| IBIS file stm32f7x2_lqfp100.ibs
[IBIS ver] 4.2
[File name] stm32f7x2_lqfp100.ibs
[File Rev] 1.1
[Date]  21-12-2016
[Source] Data Created at STMicroelectronics
[Notes]  File originated from ELDO simulations.
[Disclaimer]  This information is for modeling purpose only and is
   not guaranted.
   The information is subject to change without notice.
[Copyright] Copyright 2017 STMicroelectronics Inc.
|   Component stm32f7x2_lqfp100
[Component] stm32f7x2_lqfp100
[Manufacturer] STMicroelectronics
[Package]
| variable   typ   min   max
R_pkg   0.0   0.0   0.0
L_pkg   0.0H   0.0H   0.0H
C_pkg   0.0F   0.0F   0.0F
[Pin]  signal_name   model_name   R_pin   L_pin   C_pin
1 PE2 io8p_arsudq_ft 132.430E-3 7.034E-9 135.000E-15
2 PE3 io8p_arsudq_ft 133.348E-3 6.765E-9 19.500E-15
3 PE4 io8p_arsudq_ft 128.973E-3 6.495E-9 10.400E-15
4 PE5 io8p_arsudq_ft 125.345E-3 6.206E-9 5.240E-15
5 PE6 io8p_arsudq_ft 120.515E-3 5.991E-9 7.820E-15
6 VBAT power 120.471E-3 5.950E-9 6.530E-15
7 PC13 io8p_arwsudq_ft_v33 117.881E-3 5.783E-9 6.230E-15
8 PC14-OSC32_IN io8p_arwsudq_ft_v33 117.279E-3 5.654E-9 3.110E-15
9 PC15-OSC32_OUT io8p_arwsudq_ft 115.548E-3 5.548E-9 1.390E-15
10 VSS gnd 114.996E-3 5.434E-9 2.920E-15
11 VDD power 112.976E-3 5.296E-9 3.560E-15
12 PH0-OSC_IN io8p_arsudq_ft 111.323E-3 5.231E-9 4.780E-15
13 PH1-OSC_OUT io8p_arsudq_ft 109.217E-3 5.142E-9 8.660E-15
14 NRST ioreset_ft_v33 110.664E-3 5.180E-9 9.030E-15
15 PC0 io8p_ar3wsudq_ft 110.608E-3 5.192E-9 7.980E-15
16 PC1 io8p_ar3wsudq_ft_v33 111.326E-3 5.252E-9 10.300E-15
17 PC2 io8p_ar3wsudq_ft 114.420E-3 5.345E-9 7.000E-15
18 PC3 io8p_ar3wsudq_ft 114.363E-3 5.454E-9 8.650E-15
19 VSSA gnd 117.564E-3 5.621E-9 7.825E-15
20 VREF+ power 119.905E-3 5.800E-9 229.000E-18
21 VDDA power 122.312E-3 5.963E-9 1.050E-15
22 PA0-WKUP io8p_ar3wsudq_ft_v33 125.384E-3 6.187E-9 812.000E-18
23 PA1 io8p_ar3wsudq_ft 129.702E-3 6.485E-9 3.820E-15
24 PA2 io8p_ar3wsudq_ft_v33 132.290E-3 6.715E-9 6.800E-15
25 PA3 io8p_ar3wsudq_ft 132.955E-3 7.014E-9 16.700E-15
26 VSS gnd 133.943E-3 7.050E-9 17.500E-15
27 VDD power 134.958E-3 6.804E-9 12.700E-15
28 PA4 io8p_ar3wsudq_ft 130.511E-3 6.528E-9 9.830E-15
29 PA5 io8p_ar3wsudq_ft 125.387E-3 6.245E-9 6.070E-15
30 PA6 io8p_ar3wsudq_ft 124.989E-3 6.108E-9 577.000E-18
31 PA7 io8p_ar3wsudq_ft 121.784E-3 5.890E-9 1.520E-15
32 PC4 io8p_ar3wsudq_ft 119.149E-3 5.716E-9 5.440E-15
33 PC5 io8p_ar3wsudq_ft 116.375E-3 5.556E-9 4.100E-15
34 PB0 io8p_ar3wsudq_ft 113.279E-3 5.415E-9 3.690E-15
35 PB1 io8p_ar3wsudq_ft 112.727E-3 5.358E-9 3.895E-15
36 PB2 io8p_ar3wsudq_ft 112.271E-3 5.272E-9 1.660E-15
37 PE7 io8p_arsudq_ft 111.816E-3 5.238E-9 7.920E-15
38 PE8 io8p_arsudq_ft 110.999E-3 5.184E-9 9.900E-15
39 PE9 io8p_arsudq_ft 114.589E-3 5.299E-9 7.910E-15
40 PE10 io8p_arsudq_ft 114.461E-3 5.333E-9 7.940E-15
41 PE11 io8p_arsudq_ft 115.350E-3 5.424E-9 4.180E-15
42 PE12 io8p_arsudq_ft 116.979E-3 5.533E-9 6.060E-15
43 PE13 io8p_arsudq_ft 120.185E-3 5.698E-9 5.120E-15
44 PE14 io8p_arsudq_ft 122.587E-3 5.871E-9 4.740E-15
45 PE15 io8p_ar3wsudq_ft 126.303E-3 6.069E-9 11.600E-15
46 PB10 io8p_arsudq_i2c_ft 129.715E-3 6.277E-9 9.910E-15
47 PB11 io8p_arsudq_i2c_ft 133.373E-3 6.508E-9 5.080E-15
48 VCAP_1 power 137.888E-3 6.857E-9 5.470E-15
49 VSS gnd 131.554E-3 6.802E-9 4.180E-15
50 VDD power 132.348E-3 7.042E-9 11.900E-15
51 PB12 io8usb_id_otg_ft 131.768E-3 7.008E-9 16.200E-15
52 PB13 io8usb_vbus_otg_ft 131.784E-3 6.751E-9 2.150E-15
53 PB14 io8usb_lsfs_otg_ft 129.151E-3 6.483E-9 9.175E-15
54 PB15 io8usb_lsfs_otg_ft 125.191E-3 6.202E-9 5.663E-15
55 PD8 io8p_arsudq_ft 121.530E-3 5.986E-9 3.690E-15
56 PD9 io8p_arsudq_ft 118.874E-3 5.807E-9 7.430E-15
57 PD10 io8p_arsudq_ft 115.870E-3 5.635E-9 10.600E-15
58 PD11 io8p_arsudq_ft 113.226E-3 5.471E-9 5.760E-15
59 PD12 io8p_arsudq_ft 111.782E-3 5.354E-9 6.530E-15
60 PD13 io8p_arsudq_ft 110.713E-3 5.276E-9 11.400E-15
61 PD14 io8p_arsudq_ft 110.052E-3 5.204E-9 13.200E-15
62 PD15 io8p_arsudq_ft 109.954E-3 5.180E-9 14.600E-15
63 PC6 io8p_arsudq_ft 109.780E-3 5.154E-9 7.250E-15
64 PC7 io8p_arsudq_ft 112.446E-3 5.258E-9 359.000E-18
65 PC8 io8p_arsudq_ft 113.596E-3 5.332E-9 658.000E-18
66 PC9 io8p_arsudq_i2c_ft 115.707E-3 5.466E-9 508.500E-18
67 PA8 io8p_arsudq_i2c_ft 116.952E-3 5.598E-9 583.250E-18
68 PA9 io8usb_vbus_otg_ft 119.043E-3 5.762E-9 545.875E-18
69 PA10 io8usb_id_otg_ft 120.674E-3 5.880E-9 13.900E-15
70 PA11 io8usb_lsfs_otg_ft 124.659E-3 6.108E-9 25.000E-15
71 PA12 io8usb_lsfs_otg_ft 124.407E-3 6.161E-9 39.900E-15
72 PA13 io8p_arsudq_ft 130.156E-3 6.404E-9 302.000E-15
73 VCAP_2 power 135.110E-3 6.824E-9 155.000E-15
74 VSS gnd 139.402E-3 7.077E-9 155.000E-15
75 VDD power 133.554E-3 7.056E-9 39.000E-15
76 PA14 io8p_arsudq_ft 135.295E-3 7.104E-9 16.300E-15
77 PA15 io8p_arsudq_ft 132.514E-3 6.836E-9 9.760E-15
78 PC10 io8p_arsudq_ft 133.482E-3 6.641E-9 9.300E-15
79 PC11 io8p_arsudq_ft 128.366E-3 6.341E-9 5.420E-15
80 PC12 io8p_arsudq_ft 124.282E-3 6.092E-9 1.180E-15
81 PD0 io8p_arsudq_ft 121.841E-3 5.917E-9 5.460E-15
82 PD1 io8p_arsudq_ft 118.487E-3 5.728E-9 7.000E-15
83 PD2 io8p_arsudq_ft 117.180E-3 5.573E-9 6.060E-15
84 PD3 io8p_arsudq_ft 113.501E-3 5.422E-9 5.450E-15
85 PD4 io8p_arsudq_ft 113.789E-3 5.344E-9 529.000E-18
86 PD5 io8p_arsudq_ft 110.806E-3 5.256E-9 2.990E-15
87 PD6 io8p_arsudq_ft 110.442E-3 5.246E-9 2.060E-15
88 PD7 io8p_arsudq_ft 111.525E-3 5.178E-9 5.680E-15
89 PB3 io8p_arsudq_ft 111.144E-3 5.223E-9 9.910E-15
90 PB4 io8p_arsudq_ft 113.222E-3 5.310E-9 9.050E-15
91 PB5 io8p_ar3wsudq_ft 113.323E-3 5.401E-9 12.900E-15
92 PB6 io8p_arsudq_i2c_ft 115.849E-3 5.519E-9 12.600E-15
93 PB7 io8p_arsudq_i2c_ft 117.578E-3 5.673E-9 6.140E-15
94 BOOT0 vpp_test_hv 118.982E-3 5.802E-9 9.370E-15
95 PB8 io8p_arsudq_i2c_ft 121.886E-3 5.962E-9 7.755E-15
96 PB9 io8p_arsudq_i2c_ft 126.276E-3 6.158E-9 8.563E-15
97 PE0 io8p_arsudq_ft 128.749E-3 6.367E-9 8.159E-15
98 PE1 io8p_arsudq_ft 133.288E-3 6.700E-9 1.030E-15
99 VSS gnd 132.230E-3 6.844E-9 4.410E-15
100 VDD power 132.277E-3 7.052E-9 17.100E-15
[Diff Pin]   inv_pin   vdiff   tdelay_typ  tdelay_min  tdelay_max
53   54   NA   NA   NA   NA
70   71   NA   NA   NA   NA
[Model Selector] io8p_ar3wsudq_ft
io8p00_ar3wsudq_ft_pd_lv  "SPEED00 1P8V, PD=40kOhm"
io8p00_ar3wsudq_ft_pu_lv  "SPEED00 1P8V, PU=40kOhm"
io8p00_ar3wsudq_ft_lv  "SPEED00 1P8V"
io8p01_ar3wsudq_ft_pd_lv  "SPEED01 1P8V, PD=40kOhm"
io8p01_ar3wsudq_ft_pu_lv  "SPEED01 1P8V, PU=40kOhm"
io8p01_ar3wsudq_ft_lv  "SPEED01 1P8V"
io8p10_ar3wsudq_ft_pd_lv  "SPEED10 1P8V, PD=40kOhm"
io8p10_ar3wsudq_ft_pu_lv  "SPEED10 1P8V, PU=40kOhm"
io8p10_ar3wsudq_ft_lv  "SPEED10 1P8V"
io8p11_ar3wsudq_ft_pd_lv  "SPEED11 1P8V, PD=40kOhm"
io8p11_ar3wsudq_ft_pu_lv  "SPEED11 1P8V, PU=40kOhm"
io8p11_ar3wsudq_ft_lv  "SPEED11 1P8V"
io8p00_ar3wsudq_ft_pd  "SPEED00, PD=40kOhm"
io8p00_ar3wsudq_ft_pu  "SPEED00, PU=40kOhm"
io8p00_ar3wsudq_ft  "SPEED00"
io8p01_ar3wsudq_ft_pd  "SPEED01, PD=40kOhm"
io8p01_ar3wsudq_ft_pu  "SPEED01, PU=40kOhm"
io8p01_ar3wsudq_ft  "SPEED01"
io8p10_ar3wsudq_ft_pd  "SPEED10, PD=40kOhm"
io8p10_ar3wsudq_ft_pu  "SPEED10, PU=40kOhm"
io8p10_ar3wsudq_ft  "SPEED10"
io8p11_ar3wsudq_ft_pd  "SPEED11, PD=40kOhm"
io8p11_ar3wsudq_ft_pu  "SPEED11, PU=40kOhm"
io8p11_ar3wsudq_ft  "SPEED11"
[Model Selector] io8p_ar3wsudq_ft_v33
io8p00_ar3wsudq_ft_v33_pd_lv  "SPEED00 1P8V, PD=40kOhm"
io8p00_ar3wsudq_ft_v33_pu_lv  "SPEED00 1P8V, PU=40kOhm"
io8p00_ar3wsudq_ft_v33_lv  "SPEED00 1P8V"
io8p01_ar3wsudq_ft_v33_pd_lv  "SPEED01 1P8V, PD=40kOhm"
io8p01_ar3wsudq_ft_v33_pu_lv  "SPEED01 1P8V, PU=40kOhm"
io8p01_ar3wsudq_ft_v33_lv  "SPEED01 1P8V"
io8p10_ar3wsudq_ft_v33_pd_lv  "SPEED10 1P8V, PD=40kOhm"
io8p10_ar3wsudq_ft_v33_pu_lv  "SPEED10 1P8V, PU=40kOhm"
io8p10_ar3wsudq_ft_v33_lv  "SPEED10 1P8V"
io8p11_ar3wsudq_ft_v33_pd_lv  "SPEED11 1P8V, PD=40kOhm"
io8p11_ar3wsudq_ft_v33_pu_lv  "SPEED11 1P8V, PU=40kOhm"
io8p11_ar3wsudq_ft_v33_lv  "SPEED11 1P8V"
io8p00_ar3wsudq_ft_v33_pd  "SPEED00, PD=40kOhm"
io8p00_ar3wsudq_ft_v33_pu  "SPEED00, PU=40kOhm"
io8p00_ar3wsudq_ft_v33  "SPEED00"
io8p01_ar3wsudq_ft_v33_pd  "SPEED01, PD=40kOhm"
io8p01_ar3wsudq_ft_v33_pu  "SPEED01, PU=40kOhm"
io8p01_ar3wsudq_ft_v33  "SPEED01"
io8p10_ar3wsudq_ft_v33_pd  "SPEED10, PD=40kOhm"
io8p10_ar3wsudq_ft_v33_pu  "SPEED10, PU=40kOhm"
io8p10_ar3wsudq_ft_v33  "SPEED10"
io8p11_ar3wsudq_ft_v33_pd  "SPEED11, PD=40kOhm"
io8p11_ar3wsudq_ft_v33_pu  "SPEED11, PU=40kOhm"
io8p11_ar3wsudq_ft_v33  "SPEED11"
[Model Selector] io8p_arsudq_ft
io8p00_arsudq_ft_pd_lv  "SPEED00 1P8V, PD=40kOhm"
io8p00_arsudq_ft_pu_lv  "SPEED00 1P8V, PU=40kOhm"
io8p00_arsudq_ft_lv  "SPEED00 1P8V"
io8p01_arsudq_ft_pd_lv  "SPEED01 1P8V, PD=40kOhm"
io8p01_arsudq_ft_pu_lv  "SPEED01 1P8V, PU=40kOhm"
io8p01_arsudq_ft_lv  "SPEED01 1P8V"
io8p10_arsudq_ft_pd_lv  "SPEED10 1P8V, PD=40kOhm"
io8p10_arsudq_ft_pu_lv  "SPEED10 1P8V, PU=40kOhm"
io8p10_arsudq_ft_lv  "SPEED10 1P8V"
io8p11_arsudq_ft_pd_lv  "SPEED11 1P8V, PD=40kOhm"
io8p11_arsudq_ft_pu_lv  "SPEED11 1P8V, PU=40kOhm"
io8p11_arsudq_ft_lv  "SPEED11 1P8V"
io8p00_arsudq_ft_pd  "SPEED00, PD=40kOhm"
io8p00_arsudq_ft_pu  "SPEED00, PU=40kOhm"
io8p00_arsudq_ft  "SPEED00"
io8p01_arsudq_ft_pd  "SPEED01, PD=40kOhm"
io8p01_arsudq_ft_pu  "SPEED01, PU=40kOhm"
io8p01_arsudq_ft  "SPEED01"
io8p10_arsudq_ft_pd  "SPEED10, PD=40kOhm"
io8p10_arsudq_ft_pu  "SPEED10, PU=40kOhm"
io8p10_arsudq_ft  "SPEED10"
io8p11_arsudq_ft_pd  "SPEED11, PD=40kOhm"
io8p11_arsudq_ft_pu  "SPEED11, PU=40kOhm"
io8p11_arsudq_ft  "SPEED11"
[Model Selector] io8p_arsudq_i2c_ft
io8prog_1v8_i2c_pd  "5V Tol GPIO 1.8V range i2c functionality with pull down"
io8prog_1v8_i2c_pu  "5V Tol GPIO 1.8V range i2c functionality with pull up"
io8prog_1v8_i2c  "5V Tol GPIO 1.8V range i2c functionality"
io8prog_3v3_i2c_pd  "5V Tol GPIO 3.3V range i2c functionality with pull down"
io8prog_3v3_i2c_pu  "5V Tol GPIO 3.3V range i2c functionality with pull up"
io8prog_3v3_i2c  "5V Tol GPIO 3.3V range i2c functionality"
io8prog_1v8_pd_00  "5V Tol GPIO 1.8V range with pd speed 00"
io8prog_1v8_pu_00  "5V Tol GPIO 1.8V range with pu speed 00"
io8prog_1v8_00  "5V Tol GPIO 1.8V range speed 00"
io8prog_3v3_pd_00  "5V Tol GPIO 3.3V range with pd speed 00"
io8prog_3v3_pu_00  "5V Tol GPIO 3.3V range with pu speed 00"
io8prog_3v3_00  "5V Tol GPIO 3.3V range speed 00"
io8prog_1v8_pd_01  "5V Tol GPIO 1.8V range with pd speed 01"
io8prog_1v8_pu_01  "5V Tol GPIO 1.8V range with pu speed 01"
io8prog_1v8_01  "5V Tol GPIO 1.8V range speed 01"
io8prog_3v3_pd_01  "5V Tol GPIO 3.3V range with pd speed 01"
io8prog_3v3_pu_01  "5V Tol GPIO 3.3V range with pu speed 01"
io8prog_3v3_01  "5V Tol GPIO 3.3V range speed 01"
io8prog_1v8_pd_10  "5V Tol GPIO 1.8V range with pd speed 10"
io8prog_1v8_pu_10  "5V Tol GPIO 1.8V range with pu speed 10"
io8prog_1v8_10  "5V Tol GPIO 1.8V range speed 10"
io8prog_3v3_pd_10  "5V Tol GPIO 3.3V range with pd speed 10"
io8prog_3v3_pu_10  "5V Tol GPIO 3.3V range with pu speed 10"
io8prog_3v3_10  "5V Tol GPIO 3.3V range speed 10"
io8prog_1v8_pd_11  "5V Tol GPIO 1.8V range with pd speed 11"
io8prog_1v8_pu_11  "5V Tol GPIO 1.8V range with pu speed 11"
io8prog_1v8_11  "5V Tol GPIO 1.8V range speed 11"
io8prog_3v3_pd_11  "5V Tol GPIO 3.3V range with pd speed 11"
io8prog_3v3_pu_11  "5V Tol GPIO 3.3V range with pu speed 11"
io8prog_3v3_11  "5V Tol GPIO 3.3V range speed 11"
[Model Selector] io8p_arwsudq_ft
io8p00_arwsudq_ft_pd_lv  "SPEED00 1P8V, PD=40kOhm"
io8p00_arwsudq_ft_pu_lv  "SPEED00 1P8V, PU=40kOhm"
io8p00_arwsudq_ft_lv  "SPEED00 1P8V"
io8p01_arwsudq_ft_pd_lv  "SPEED01 1P8V, PD=40kOhm"
io8p01_arwsudq_ft_pu_lv  "SPEED01 1P8V, PU=40kOhm"
io8p01_arwsudq_ft_lv  "SPEED01 1P8V"
io8p10_arwsudq_ft_pd_lv  "SPEED10 1P8V, PD=40kOhm"
io8p10_arwsudq_ft_pu_lv  "SPEED10 1P8V, PU=40kOhm"
io8p10_arwsudq_ft_lv  "SPEED10 1P8V"
io8p11_arwsudq_ft_pd_lv  "SPEED11 1P8V, PD=40kOhm"
io8p11_arwsudq_ft_pu_lv  "SPEED11 1P8V, PU=40kOhm"
io8p11_arwsudq_ft_lv  "SPEED11 1P8V"
io8p00_arwsudq_ft_pd  "SPEED00, PD=40kOhm"
io8p00_arwsudq_ft_pu  "SPEED00, PU=40kOhm"
io8p00_arwsudq_ft  "SPEED00"
io8p01_arwsudq_ft_pd  "SPEED01, PD=40kOhm"
io8p01_arwsudq_ft_pu  "SPEED01, PU=40kOhm"
io8p01_arwsudq_ft  "SPEED01"
io8p10_arwsudq_ft_pd  "SPEED10, PD=40kOhm"
io8p10_arwsudq_ft_pu  "SPEED10, PU=40kOhm"
io8p10_arwsudq_ft  "SPEED10"
io8p11_arwsudq_ft_pd  "SPEED11, PD=40kOhm"
io8p11_arwsudq_ft_pu  "SPEED11, PU=40kOhm"
io8p11_arwsudq_ft  "SPEED11"
[Model Selector] io8p_arwsudq_ft_v33
io8p00_arwsudq_ft_v33_pd_lv  "SPEED00 1P8V, PD=40kOhm"
io8p00_arwsudq_ft_v33_pu_lv  "SPEED00 1P8V, PU=40kOhm"
io8p00_arwsudq_ft_v33_lv  "SPEED00 1P8V"
io8p01_arwsudq_ft_v33_pd_lv  "SPEED01 1P8V, PD=40kOhm"
io8p01_arwsudq_ft_v33_pu_lv  "SPEED01 1P8V, PU=40kOhm"
io8p01_arwsudq_ft_v33_lv  "SPEED01 1P8V"
io8p10_arwsudq_ft_v33_pd_lv  "SPEED10 1P8V, PD=40kOhm"
io8p10_arwsudq_ft_v33_pu_lv  "SPEED10 1P8V, PU=40kOhm"
io8p10_arwsudq_ft_v33_lv  "SPEED10 1P8V"
io8p11_arwsudq_ft_v33_pd_lv  "SPEED11 1P8V, PD=40kOhm"
io8p11_arwsudq_ft_v33_pu_lv  "SPEED11 1P8V, PU=40kOhm"
io8p11_arwsudq_ft_v33_lv  "SPEED11 1P8V"
io8p00_arwsudq_ft_v33_pd  "SPEED00, PD=40kOhm"
io8p00_arwsudq_ft_v33_pu  "SPEED00, PU=40kOhm"
io8p00_arwsudq_ft_v33  "SPEED00"
io8p01_arwsudq_ft_v33_pd  "SPEED01, PD=40kOhm"
io8p01_arwsudq_ft_v33_pu  "SPEED01, PU=40kOhm"
io8p01_arwsudq_ft_v33  "SPEED01"
io8p10_arwsudq_ft_v33_pd  "SPEED10, PD=40kOhm"
io8p10_arwsudq_ft_v33_pu  "SPEED10, PU=40kOhm"
io8p10_arwsudq_ft_v33  "SPEED10"
io8p11_arwsudq_ft_v33_pd  "SPEED11, PD=40kOhm"
io8p11_arwsudq_ft_v33_pu  "SPEED11, PU=40kOhm"
io8p11_arwsudq_ft_v33  "SPEED11"
[Model Selector] io8usb_id_otg_ft
io8p00_id_otg_ft_pd_lv  "SPEED00 1P8V, PD=14kOhm"
io8p00_id_otg_ft_pu_lv  "SPEED00 1P8V, PU=14kOhm"
io8p00_id_otg_ft_lv  "SPEED00 1P8V"
io8p01_id_otg_ft_pd_lv  "SPEED01 1P8V, PD=14kOhm"
io8p01_id_otg_ft_pu_lv  "SPEED01 1P8V, PU=14kOhm"
io8p01_id_otg_ft_lv  "SPEED01 1P8V"
io8p10_id_otg_ft_pd_lv  "SPEED10 1P8V, PD=14kOhm"
io8p10_id_otg_ft_pu_lv  "SPEED10 1P8V, PU=14kOhm"
io8p10_id_otg_ft_lv  "SPEED10 1P8V"
io8p11_id_otg_ft_pd_lv  "SPEED11 1P8V, PD=14kOhm"
io8p11_id_otg_ft_pu_lv  "SPEED11 1P8V, PU=14kOhm"
io8p11_id_otg_ft_lv  "SPEED11 1P8V"
io8p00_id_otg_ft_pd  "SPEED00, PD=14kOhm"
io8p00_id_otg_ft_pu  "SPEED00, PU=14kOhm"
io8p00_id_otg_ft  "SPEED00"
io8p01_id_otg_ft_pd  "SPEED01, PD=14kOhm"
io8p01_id_otg_ft_pu  "SPEED01, PU=14kOhm"
io8p01_id_otg_ft  "SPEED01"
io8p10_id_otg_ft_pd  "SPEED10, PD=14kOhm"
io8p10_id_otg_ft_pu  "SPEED10, PU=14kOhm"
io8p10_id_otg_ft  "SPEED10"
io8p11_id_otg_ft_pd  "SPEED11, PD=14kOhm"
io8p11_id_otg_ft_pu  "SPEED11, PU=14kOhm"
io8p11_id_otg_ft  "SPEED11"
[Model Selector] io8usb_lsfs_otg_ft
io8usb_ls_otg_ft_dpdn_pd  "LS USB DP/DN IO + PD=20kOhm"
io8usb_ls_otg_ft_dpdn_pupu2  "LS USB DP/DN IO + PU/PU2=2.2kOhm"
io8usb_ls_otg_ft_dpdn_pu2  "LS USB DP/DN IO + PU2=1.2kOhm"
io8usb_ls_otg_ft_dpdn_pu  "LS USB DP/DN IO + PU=1.2kOhm"
io8usb_ls_otg_ft_dpdn  "LS USB DP/DN IO"
io8usb_fs_otg_ft_dpdn_pd  "HS USB DP/DN IO + PD=20kOhm"
io8usb_fs_otg_ft_dpdn_pupu2  "HS USB DP/DN IO + PU/PU2=2.2kOhm"
io8usb_fs_otg_ft_dpdn_pu2  "HS USB DP/DN IO + PU2=1.2kOhm"
io8usb_fs_otg_ft_dpdn_pu  "HS USB DP/DN IO + PU=1.2kOhm"
io8usb_fs_otg_ft_dpdn  "HS USB DP/DN IO"
io8p00_lsfs_otg_ft_pd_lv  "SPEED00 1P8V, PD=40kOhm"
io8p00_lsfs_otg_ft_pu_lv  "SPEED00 1P8V, PU=40kOhm"
io8p00_lsfs_otg_ft_lv  "SPEED00 1P8V"
io8p01_lsfs_otg_ft_pd_lv  "SPEED01 1P8V, PD=40kOhm"
io8p01_lsfs_otg_ft_pu_lv  "SPEED01 1P8V, PU=40kOhm"
io8p01_lsfs_otg_ft_lv  "SPEED01 1P8V"
io8p10_lsfs_otg_ft_pd_lv  "SPEED10 1P8V, PD=40kOhm"
io8p10_lsfs_otg_ft_pu_lv  "SPEED10 1P8V, PU=40kOhm"
io8p10_lsfs_otg_ft_lv  "SPEED10 1P8V"
io8p11_lsfs_otg_ft_pd_lv  "SPEED11 1P8V, PD=40kOhm"
io8p11_lsfs_otg_ft_pu_lv  "SPEED11 1P8V, PU=40kOhm"
io8p11_lsfs_otg_ft_lv  "SPEED11 1P8V"
io8p00_lsfs_otg_ft_pd  "SPEED00, PD=40kOhm"
io8p00_lsfs_otg_ft_pu  "SPEED00, PU=40kOhm"
io8p00_lsfs_otg_ft  "SPEED00"
io8p01_lsfs_otg_ft_pd  "SPEED01, PD=40kOhm"
io8p01_lsfs_otg_ft_pu  "SPEED01, PU=40kOhm"
io8p01_lsfs_otg_ft  "SPEED01"
io8p10_lsfs_otg_ft_pd  "SPEED10, PD=40kOhm"
io8p10_lsfs_otg_ft_pu  "SPEED10, PU=40kOhm"
io8p10_lsfs_otg_ft  "SPEED10"
io8p11_lsfs_otg_ft_pd  "SPEED11, PD=40kOhm"
io8p11_lsfs_otg_ft_pu  "SPEED11, PU=40kOhm"
io8p11_lsfs_otg_ft  "SPEED11"
[Model Selector] io8usb_vbus_otg_ft
io8psenb_vbus_otg_ft  "VBUS PULSE, SENSE VB"
io8psenab_vbus_otg_ft  "VBUS PULSE, SENSE VA and VB"
io8psena_vbus_otg_ft  "VBUS PULSE, SENSE VA"
io8psen_vbus_otg_ft  "VBUS PULSE"
io8p00_vbus_otg_ft_pd_lv  "SPEED00 1P8V, PD=40kOhm"
io8p00_vbus_otg_ft_pu_lv  "SPEED00 1P8V, PU=40kOhm"
io8p00_vbus_otg_ft_lv  "SPEED00 1P8V"
io8p01_vbus_otg_ft_pd_lv  "SPEED01 1P8V, PD=40kOhm"
io8p01_vbus_otg_ft_pu_lv  "SPEED01 1P8V, PU=40kOhm"
io8p01_vbus_otg_ft_lv  "SPEED01 1P8V"
io8p10_vbus_otg_ft_pd_lv  "SPEED10 1P8V, PD=40kOhm"
io8p10_vbus_otg_ft_pu_lv  "SPEED10 1P8V, PU=40kOhm"
io8p10_vbus_otg_ft_lv  "SPEED10 1P8V"
io8p11_vbus_otg_ft_pd_lv  "SPEED11 1P8V, PD=40kOhm"
io8p11_vbus_otg_ft_pu_lv  "SPEED11 1P8V, PU=40kOhm"
io8p11_vbus_otg_ft_lv  "SPEED11 1P8V"
io8p00_vbus_otg_ft_pd  "SPEED00, PD=40kOhm"
io8p00_vbus_otg_ft_pu  "SPEED00, PU=40kOhm"
io8p00_vbus_otg_ft  "SPEED00"
io8p01_vbus_otg_ft_pd  "SPEED01, PD=40kOhm"
io8p01_vbus_otg_ft_pu  "SPEED01, PU=40kOhm"
io8p01_vbus_otg_ft  "SPEED01"
io8p10_vbus_otg_ft_pd  "SPEED10, PD=40kOhm"
io8p10_vbus_otg_ft_pu  "SPEED10, PU=40kOhm"
io8p10_vbus_otg_ft  "SPEED10"
io8p11_vbus_otg_ft_pd  "SPEED11, PD=40kOhm"
io8p11_vbus_otg_ft_pu  "SPEED11, PU=40kOhm"
io8p11_vbus_otg_ft  "SPEED11"
[Model Selector] ioreset_ft_v33
ioreset_ft_v33_pu_lv  "IORESET 1P8V + PU=40kOhm"
ioreset_ft_v33_nopu_lv  "IORESET 1P8V"
ioreset_ft_v33_pu  "IORESET + PU=40kOhm"
ioreset_ft_v33_nopu  "IORESET"
[Model Selector] vpp_test_hv
vpp_test_hv_2p4  "Input Buffer 1P8V"
vpp_test_hv_3p3  "Input Buffer"
| Models and submodels in the file (242): io8p00_ar3wsudq_ft_pd_lv (I/O), io8p00_ar3wsudq_ft_pu_lv (I/O), io8p00_ar3wsudq_ft_lv (I/O), io8p01_ar3wsudq_ft_pd_lv (I/O), io8p01_ar3wsudq_ft_pu_lv (I/O), io8p01_ar3wsudq_ft_lv (I/O), io8p10_ar3wsudq_ft_pd_lv (I/O), io8p10_ar3wsudq_ft_pu_lv (I/O), io8p10_ar3wsudq_ft_lv (I/O), io8p11_ar3wsudq_ft_pd_lv (I/O), io8p11_ar3wsudq_ft_pu_lv (I/O), io8p11_ar3wsudq_ft_lv (I/O), io8p00_ar3wsudq_ft_pd (I/O), io8p00_ar3wsudq_ft_pu (I/O), io8p00_ar3wsudq_ft (I/O), io8p01_ar3wsudq_ft_pd (I/O), io8p01_ar3wsudq_ft_pu (I/O), io8p01_ar3wsudq_ft (I/O), io8p10_ar3wsudq_ft_pd (I/O), io8p10_ar3wsudq_ft_pu (I/O), io8p10_ar3wsudq_ft (I/O), io8p11_ar3wsudq_ft_pd (I/O), io8p11_ar3wsudq_ft_pu (I/O), io8p11_ar3wsudq_ft (I/O), io8p00_ar3wsudq_ft_v33_pd_lv (I/O), io8p00_ar3wsudq_ft_v33_pu_lv (I/O), io8p00_ar3wsudq_ft_v33_lv (I/O), io8p01_ar3wsudq_ft_v33_pd_lv (I/O), io8p01_ar3wsudq_ft_v33_pu_lv (I/O), io8p01_ar3wsudq_ft_v33_lv (I/O), io8p10_ar3wsudq_ft_v33_pd_lv (I/O), io8p10_ar3wsudq_ft_v33_pu_lv (I/O), io8p10_ar3wsudq_ft_v33_lv (I/O), io8p11_ar3wsudq_ft_v33_pd_lv (I/O), io8p11_ar3wsudq_ft_v33_pu_lv (I/O), io8p11_ar3wsudq_ft_v33_lv (I/O), io8p00_ar3wsudq_ft_v33_pd (I/O), io8p00_ar3wsudq_ft_v33_pu (I/O), io8p00_ar3wsudq_ft_v33 (I/O), io8p01_ar3wsudq_ft_v33_pd (I/O), io8p01_ar3wsudq_ft_v33_pu (I/O), io8p01_ar3wsudq_ft_v33 (I/O), io8p10_ar3wsudq_ft_v33_pd (I/O), io8p10_ar3wsudq_ft_v33_pu (I/O), io8p10_ar3wsudq_ft_v33 (I/O), io8p11_ar3wsudq_ft_v33_pd (I/O), io8p11_ar3wsudq_ft_v33_pu (I/O), io8p11_ar3wsudq_ft_v33 (I/O), io8p00_arsudq_ft_pd_lv (I/O), io8p00_arsudq_ft_pu_lv (I/O), io8p00_arsudq_ft_lv (I/O), io8p01_arsudq_ft_pd_lv (I/O), io8p01_arsudq_ft_pu_lv (I/O), io8p01_arsudq_ft_lv (I/O), io8p10_arsudq_ft_pd_lv (I/O), io8p10_arsudq_ft_pu_lv (I/O), io8p10_arsudq_ft_lv (I/O), io8p11_arsudq_ft_pd_lv (I/O), io8p11_arsudq_ft_pu_lv (I/O), io8p11_arsudq_ft_lv (I/O), io8p00_arsudq_ft_pd (I/O), io8p00_arsudq_ft_pu (I/O), io8p00_arsudq_ft (I/O), io8p01_arsudq_ft_pd (I/O), io8p01_arsudq_ft_pu (I/O), io8p01_arsudq_ft (I/O), io8p10_arsudq_ft_pd (I/O), io8p10_arsudq_ft_pu (I/O), io8p10_arsudq_ft (I/O), io8p11_arsudq_ft_pd (I/O), io8p11_arsudq_ft_pu (I/O), io8p11_arsudq_ft (I/O), io8prog_1v8_i2c_pd (I/O), io8prog_1v8_i2c_pu (I/O), io8prog_1v8_i2c (I/O), io8prog_3v3_i2c_pd (I/O), io8prog_3v3_i2c_pu (I/O), io8prog_3v3_i2c (I/O), io8prog_1v8_pd_00 (I/O), io8prog_1v8_pu_00 (I/O)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
